(* Logix 5000 AddOnInstructionDefinition export B256_CtoE; software revision 30.00 *)

ADD_ON_INSTRUCTION D_SHR   (* revision 1.0, vendor Ken Fischer, NSWCPD, C512 *)
// DINT bit shift right of the 32-bit argument Inp_A by Inp_B bits with paddding by zeros on the right
// Revision note:
// Rev1.0: TBD - Initial Release
VAR_IN_OUT
   Inp_A : DINT; {required}   // 64-bit Integer to be right circular rotated
END_VAR
VAR_INPUT
   Inp_B : INT; {required}   // Number of bits to shift
END_VAR
VAR_IN_OUT
   Out : DINT; {required}   // Result
END_VAR
VAR
   BSR_Cntrl : CONTROL := (LEN := 32);
   ONS : BOOL;
   Source_Bit : BOOL;
   Wrk_InpA : DINT[2];
END_VAR

ROUTINE Logic   (* ladder *)
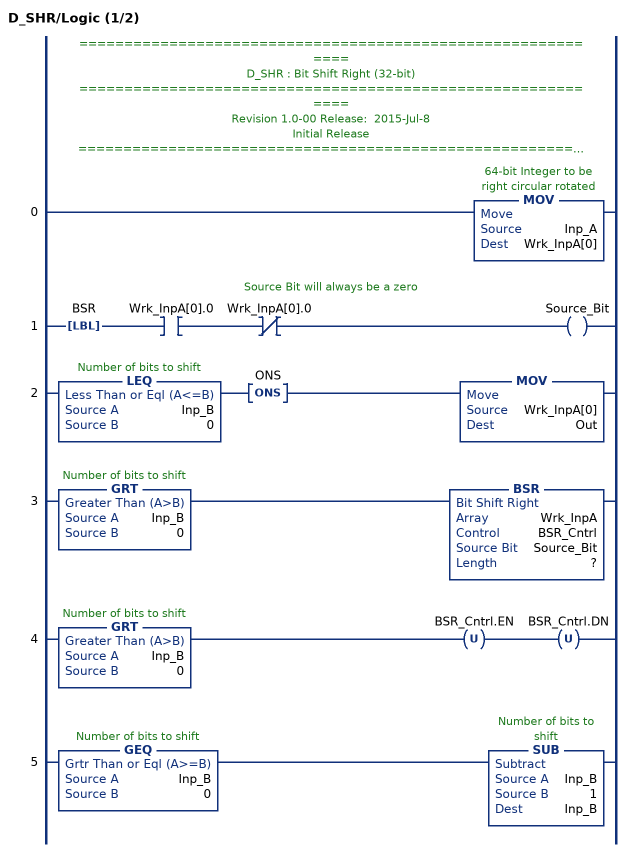
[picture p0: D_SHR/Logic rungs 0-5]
   // ============================================================
   // D_SHR : Bit Shift Right (32-bit)
   // ============================================================
   // Revision 1.0-00 Release:  2015-Jul-8
   // Initial Release
   // ============================================================
   // Performs a right bit shift of the 32-bit argument Inp_A by the
   // number of bits defined in the 16-bit argument Inp_B, with padding by zeros.
   0: MOV(Inp_A,Wrk_InpA[0]);
   // Source Bit will always be a zero
   1: LBL(BSR)XIC(Wrk_InpA[0].0)XIO(Wrk_InpA[0].0)OTE(Source_Bit);
   2: LEQ(Inp_B,0)ONS(ONS)MOV(Wrk_InpA[0],Out);
   3: GRT(Inp_B,0)BSR(Wrk_InpA,BSR_Cntrl,Source_Bit,?);
   4: GRT(Inp_B,0)OTU(BSR_Cntrl.EN)OTU(BSR_Cntrl.DN);
   5: GEQ(Inp_B,0)SUB(Inp_B,1,Inp_B);
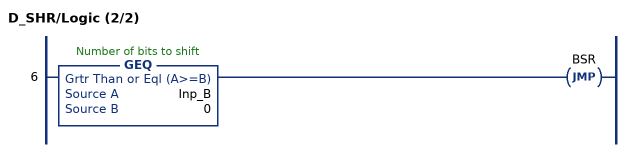
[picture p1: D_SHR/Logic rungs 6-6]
   6: GEQ(Inp_B,0)JMP(BSR);
END_ROUTINE
END_ADD_ON_INSTRUCTION

ADD_ON_INSTRUCTION D_SHL   (* revision 1.0, vendor Ken Fischer, NSWCPD, C512 *)
// DINT bit shift left of the 32-bit argument Inp_A by Inp_B bits with paddding by zeros on the right
// Revision note:
// Rev1.0: TBD - Initial Release
VAR_IN_OUT
   Inp_A : DINT; {required}   // 64-bit Integer to be right circular rotated
END_VAR
VAR_INPUT
   Inp_B : INT; {required}   // Number of bits to shift
END_VAR
VAR_IN_OUT
   Out : DINT; {required}   // Result
END_VAR
VAR
   Wrk_InpA : DINT[2];
   Source_Bit : BOOL;
   ONS : BOOL;
   BSL_Cntrl : CONTROL := (LEN := 32);
END_VAR

ROUTINE Logic   (* ladder *)
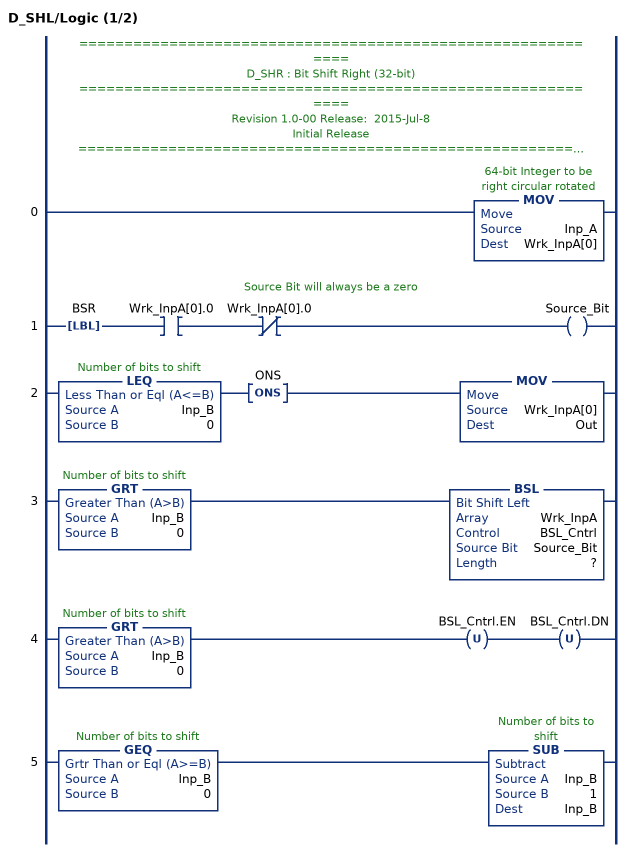
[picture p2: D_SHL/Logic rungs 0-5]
   // ============================================================
   // D_SHR : Bit Shift Right (32-bit)
   // ============================================================
   // Revision 1.0-00 Release:  2015-Jul-8
   // Initial Release
   // ============================================================
   // Performs a left bit shift of the 32-bit argument Inp_A by the
   // number of bits defined in the 16-bit argument Inp_B, with padding by zeros.
   0: MOV(Inp_A,Wrk_InpA[0]);
   // Source Bit will always be a zero
   1: LBL(BSR)XIC(Wrk_InpA[0].0)XIO(Wrk_InpA[0].0)OTE(Source_Bit);
   2: LEQ(Inp_B,0)ONS(ONS)MOV(Wrk_InpA[0],Out);
   3: GRT(Inp_B,0)BSL(Wrk_InpA,BSL_Cntrl,Source_Bit,?);
   4: GRT(Inp_B,0)OTU(BSL_Cntrl.EN)OTU(BSL_Cntrl.DN);
   5: GEQ(Inp_B,0)SUB(Inp_B,1,Inp_B);
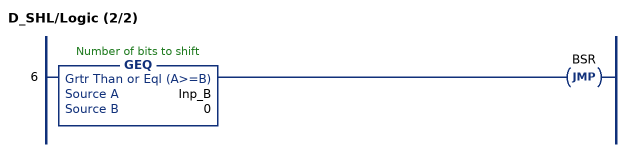
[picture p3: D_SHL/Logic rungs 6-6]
   6: GEQ(Inp_B,0)JMP(BSR);
END_ROUTINE
END_ADD_ON_INSTRUCTION

ADD_ON_INSTRUCTION B256_CtoE   (* revision 1.0 20170916, vendor Kenneth A. Fischer *)
// Convert 256-bit value using 22 12-bit pieces into 256-bit value using 32 8-bit pieces
// Revision note:
// Rev1.0: 20170916 - Initial Release
VAR_IN_OUT
   Inp_C : DINT[22]; {required}
   Out_E : DINT[32]; {required}
END_VAR
VAR
   i : INT;
   j : INT;
   TEMP1 : DINT;
   TEMP2 : DINT;
   D_SHL : D_SHL;
   D_SHR : D_SHR;
END_VAR

ROUTINE Logic   (* ladder *)
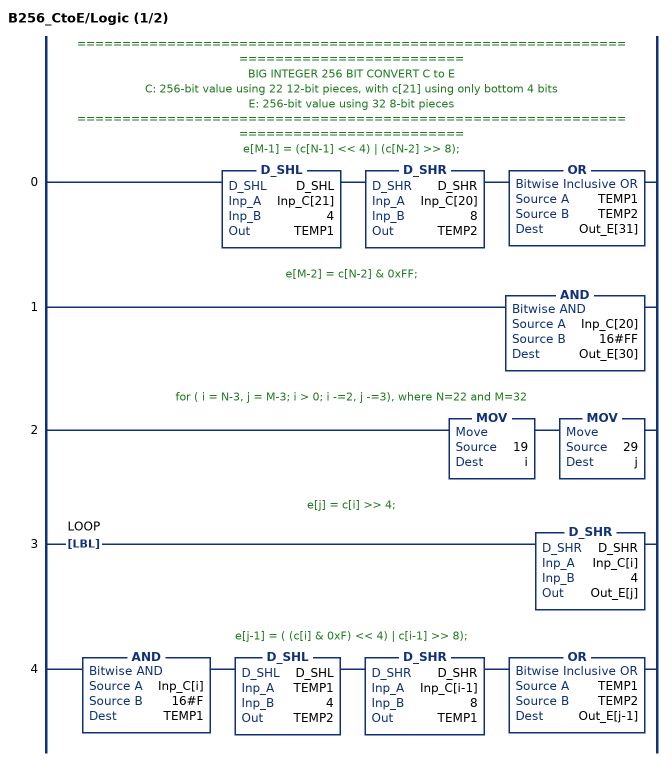
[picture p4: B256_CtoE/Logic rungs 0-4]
   // ======================================================================================
   // BIG INTEGER 256 BIT CONVERT C to E
   // C: 256-bit value using 22 12-bit pieces, with c[21] using only bottom 4 bits
   // E: 256-bit value using 32 8-bit pieces
   // ======================================================================================
   // e[M-1] = (c[N-1] << 4) | (c[N-2] >> 8);
   0: D_SHL(D_SHL,Inp_C[21],4,TEMP1)D_SHR(D_SHR,Inp_C[20],8,TEMP2)OR(TEMP1,TEMP2,Out_E[31]);
   // e[M-2] = c[N-2] & 0xFF;
   1: AND(Inp_C[20],16#FF,Out_E[30]);
   // for ( i = N-3, j = M-3; i > 0; i -=2, j -=3), where N=22 and M=32
   2: MOV(19,i)MOV(29,j);
   // e[j] = c[i] >> 4;
   3: LBL(LOOP)D_SHR(D_SHR,Inp_C[i],4,Out_E[j]);
   // e[j-1] = ( (c[i] & 0xF) << 4) | c[i-1] >> 8);
   4: AND(Inp_C[i],16#F,TEMP1)D_SHL(D_SHL,TEMP1,4,TEMP2)D_SHR(D_SHR,Inp_C[i-1],8,TEMP1)OR(TEMP1,TEMP2,Out_E[j-1]);
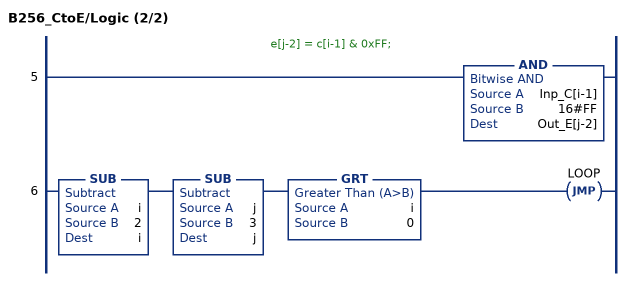
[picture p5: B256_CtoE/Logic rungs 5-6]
   // e[j-2] = c[i-1] & 0xFF;
   5: AND(Inp_C[i-1],16#FF,Out_E[j-2]);
   6: SUB(i,2,i)SUB(j,3,j)GRT(i,0)JMP(LOOP);
END_ROUTINE
END_ADD_ON_INSTRUCTION
